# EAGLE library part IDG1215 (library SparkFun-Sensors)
Invensense IDG1215 Dual-Axis 67 &deg;/s Gyro he IDG-1215 is an integrated dual-axis angular rate sensor (gyroscope). It uses InvenSense’s proprietary and patented MEMS technology with vertically driven, vibrating masses to make a functionally complete, low-cost, dual-axis angular rate sensor. All required electronics are integrated onto a single chip with the sensor. Datasheet SparkFun Products Dual Axis Gyro - IDG1215 (COM-09071) Gyro Breakout Board - IDG1215 Dual 67°/s (SEN-09093)
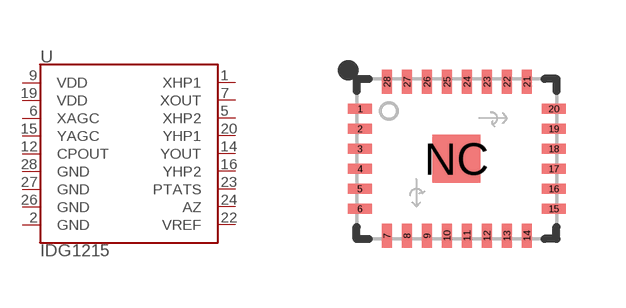
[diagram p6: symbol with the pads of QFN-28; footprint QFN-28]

Designator prefix U

## IDG1215 (PROD_ID: IC-09061; SF_ID: COM-09071)  [QFN-28]
1  XHP1
2  GND
5  XHP2
6  XAGC
7  XOUT
9  VDD
12  CPOUT
14  YOUT
15  YAGC
16  YHP2
19  VDD
20  YHP1
22  VREF
23  PTATS
24  AZ
26  GND
27  GND
28  GND

## Footprint QFN-28 (pad centres in mm)
28-Pin QFN w/ Center Pad (5 x 4 mm) Datasheet Specifications: Pin Count: 28 Dimensions: 4.0 x 5.0 x 1.15 mm Pitch: 0.5 mm Devices Using: IDG1215
smd 0.6 x 0.25: 1 -2.417,1.25; 2 -2.417,0.75; 3 -2.417,0.25; 4 -2.417,-0.25; 5 -2.417,-0.75; 6 -2.417,-1.25; 15 2.433,-1.25; 16 2.433,-0.75; 17 2.433,-0.25; 18 2.433,0.25; 19 2.433,0.75; 20 2.433,1.25
smd 0.25 x 0.6: 7 -1.742,-1.925; 8 -1.242,-1.925; 9 -0.742,-1.925; 10 -0.242,-1.925; 11 0.258,-1.925; 12 0.758,-1.925; 13 1.258,-1.925; 14 1.758,-1.925; 21 1.758,1.925; 22 1.258,1.925; 23 0.758,1.925; 24 0.258,1.925; 25 -0.242,1.925; 26 -0.742,1.925; 27 -1.242,1.925; 28 -1.742,1.925
smd 1.2 x 1.2: NC 0,0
